(* Logix 5000 DataType export; software revision 16.04 *)

TYPE AKD_Status :   // All connections to the drive ethernet module are established and data is successfully transferring.
STRUCT
   Profile_In_Progress : BOOL;   // Profile Move In Progress
   Block_In_Execution : BOOL;   // Block In Execution
   On_Target_Position : BOOL;   // On Target Position (1=Current Position Equals Last Target Position)
   General_Fault : BOOL;   // General Fault
   Current_Direction : BOOL;   // Current Motor Direction (0=Reverse, 1=Forward)
   Home_Level : BOOL;   // Level of Home Input
   Reg_Level : BOOL;   // Level of Registration Input
   Enable : BOOL;   // State of Enable Output
   Fault_Input_Fault : BOOL;   // Fault Input Active
   Fwd_Limit : BOOL;   // Forward Input Active
   Rev_Limit : BOOL;   // Reverse Input Active
   Positive_Limit : BOOL;   // Positive Software Limit Exceeded
   Negative_Limit : BOOL;   // Negative Software Limit Exceeded
   FE_Fault : BOOL;   // Following Error Fault
   Block_Fault : BOOL;   // Block Execution Fault
   Load_Complete : BOOL;   // Command Message Successfully Loaded
END_STRUCT
END_TYPE
